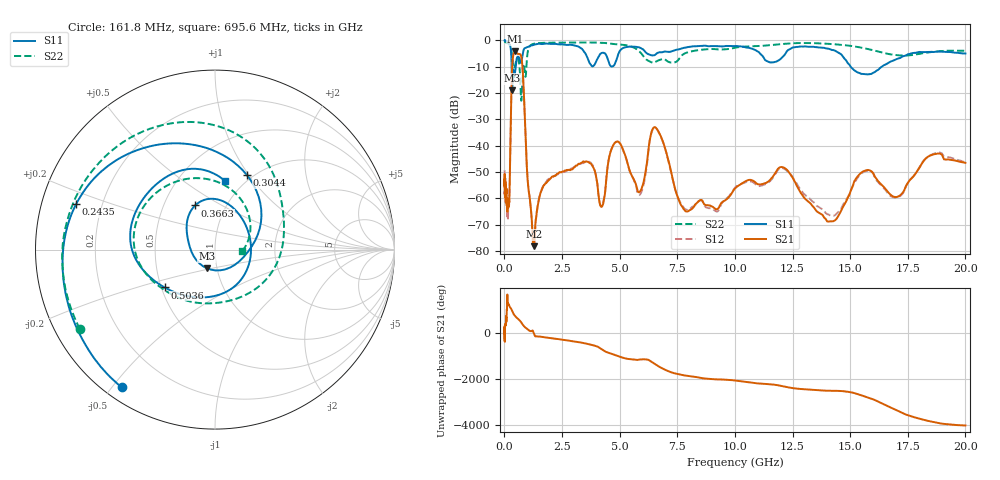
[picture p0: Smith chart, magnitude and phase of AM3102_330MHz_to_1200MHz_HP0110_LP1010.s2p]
! Date/Time: Tue, Sep 11, 2018 5:15 PM
! Network Analyzer: Agilent Technologies E8362B Rev: A.07.50.63
! Sweep from 0.010 to 20.000 GHz, 1601 Points, Sweep Type: LOG
! Power Supply: 4.949 V, 0.001 A
# Hz S DB R 50
!freq MagS11 AngS11 MagS21 AngS21 MagS12 AngS12 MagS22 AngS22
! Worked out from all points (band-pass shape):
!   1601 points, 10 MHz to 20 GHz, reference 50 ohm
!   highest |S21| = -4.12 dB at 475.7 MHz (marker M1); lowest = -78.1 dB at 1.272 GHz (marker M2)
!   |S21| within 3 dB of the highest: 358 MHz to 750.9 MHz (392.9 MHz wide, 70.9 % of centre)
!   lowest |S11| = -18.9 dB at 337.9 MHz (marker M3), VSWR 1.26, Z = 44.7 - j9.4 ohm
!   |S11| at or under -10 dB: 314.9 MHz to 493.2 MHz (178.3 MHz wide, 44.1 % of centre); 15.03 GHz to 16.37 GHz (1.345 GHz wide, 8.57 % of centre)
!   |S22| runs from -22.9 to -0.3 dB; largest |S21 - S12| = 0.011
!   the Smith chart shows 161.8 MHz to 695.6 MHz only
!   S11 on the Smith chart (normalised r, x): 161.8 MHz: 0.05, -0.53; 243.5 MHz: 0.11, +0.16; 304.4 MHz: 0.93, +0.98; 366.3 MHz: 0.72, +0.38; 503.6 MHz: 0.52, -0.25; 695.6 MHz: 0.82, +0.74
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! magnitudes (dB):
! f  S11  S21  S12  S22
! 10 MHz  0.0  -53.8  -49.3  -0.3
! 35.55 MHz  0.0  -58.3  -56.4  -0.5
! 126.4 MHz  -0.4  -64.9  -65.0  -1.0
! 161.8 MHz  -0.7  -62.7  -64.5  -1.2
! 243.5 MHz  -1.8  -48.0  -48.1  -1.8
! 304.4 MHz  -6.9  -19.5  -19.6  -3.5
! 337.9 MHz  -18.9  -9.6  -9.6  -6.5
! 366.3 MHz  -11.4  -6.6  -6.6  -8.5
! 447.2 MHz  -13.1  -4.2  -4.2  -10.0
! 475.7 MHz  -11.4  -4.1  -4.1  -9.1
! 503.6 MHz  -9.1  -4.3  -4.4  -8.0
! 695.6 MHz  -8.3  -5.3  -5.3  -16.4
! 1.272 GHz  -1.7  -78.1  -76.5  -1.3
! 1.59 GHz  -1.3  -57.4  -57.2  -0.9
! 4.23 GHz  -4.7  -63.1  -62.8  -0.9
! 4.878 GHz  -7.0  -38.4  -38.5  -1.5
! 5.652 GHz  -2.4  -53.5  -53.8  -2.9
! 6.58 GHz  -5.1  -33.2  -33.4  -8.0
! 7.845 GHz  -2.7  -64.8  -64.1  -4.8
! 12.03 GHz  -6.6  -48.1  -48.4  -1.4
! 14.07 GHz  -3.2  -68.8  -66.1  -1.3
! 20 GHz  -4.9  -46.5  -46.4  -3.9
